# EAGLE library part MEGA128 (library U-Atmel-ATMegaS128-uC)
MICROCONTROLLER 128 Kbytes FLASH 4 Kbytes SRAM 4 Kbytes EEPROM DUAL USART 8-channel 10 bit ADC Source: avr.lbr
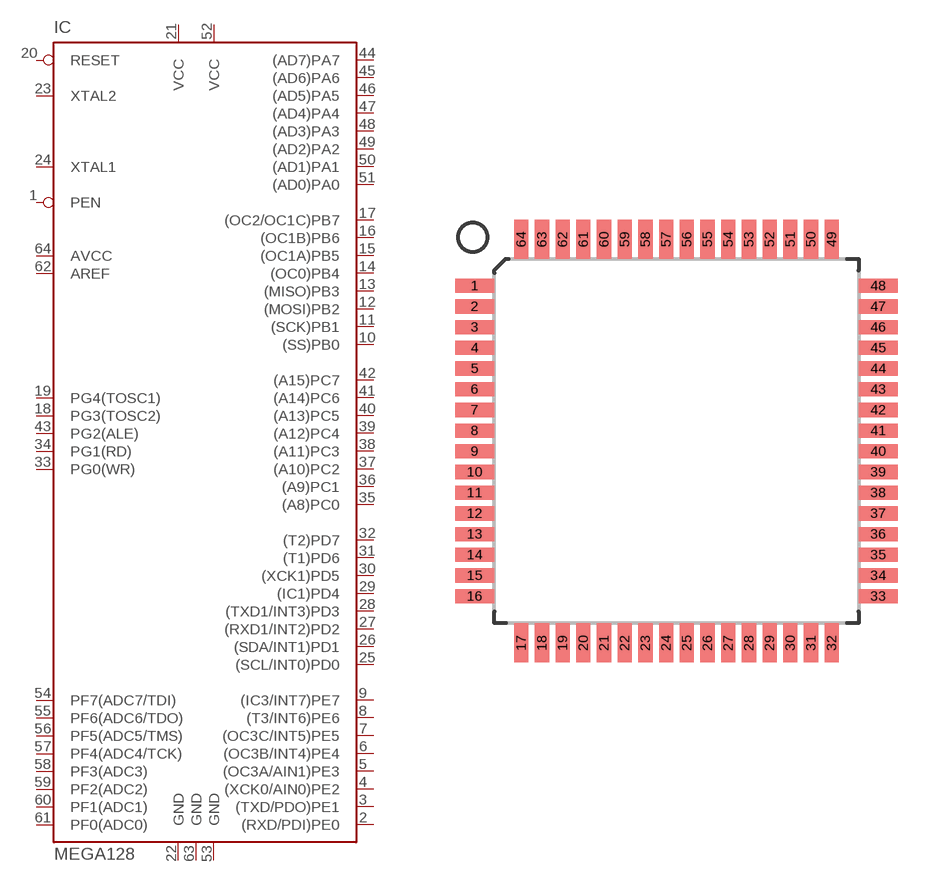
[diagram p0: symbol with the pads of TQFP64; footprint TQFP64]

Designator prefix IC

## MEGA128-A (MPN: ATMEGA128-16AU; OC_FARNELL: 9171118; OC_NEWARK: 95K7364)  [TQFP64]
1  PEN  in
2  (RXD/PDI)PE0
3  (TXD/PDO)PE1
4  (XCK0/AIN0)PE2
5  (OC3A/AIN1)PE3
6  (OC3B/INT4)PE4
7  (OC3C/INT5)PE5
8  (T3/INT6)PE6
9  (IC3/INT7)PE7
10  (SS)PB0
11  (SCK)PB1
12  (MOSI)PB2
13  (MISO)PB3
14  (OC0)PB4
15  (OC1A)PB5
16  (OC1B)PB6
17  (OC2/OC1C)PB7
18  PG3(TOSC2)
19  PG4(TOSC1)
20  RESET  in
21  VCC  pwr
22  GND  pwr
23  XTAL2  pas
24  XTAL1  pas
25  (SCL/INT0)PD0
26  (SDA/INT1)PD1
27  (RXD1/INT2)PD2
28  (TXD1/INT3)PD3
29  (IC1)PD4
30  (XCK1)PD5
31  (T1)PD6
32  (T2)PD7
33  PG0(WR)
34  PG1(RD)
35  (A8)PC0
36  (A9)PC1
37  (A10)PC2
38  (A11)PC3
39  (A12)PC4
40  (A13)PC5
41  (A14)PC6
42  (A15)PC7
43  PG2(ALE)
44  (AD7)PA7
45  (AD6)PA6
46  (AD5)PA5
47  (AD4)PA4
48  (AD3)PA3
49  (AD2)PA2
50  (AD1)PA1
51  (AD0)PA0
52  VCC  pwr
53  GND  pwr
54  PF7(ADC7/TDI)
55  PF6(ADC6/TDO)
56  PF5(ADC5/TMS)
57  PF4(ADC4/TCK)
58  PF3(ADC3)
59  PF2(ADC2)
60  PF1(ADC1)
61  PF0(ADC0)
62  AREF  pas
63  GND  pwr
64  AVCC  pwr

## Footprint TQFP64 (pad centres in mm)
Thin Plasic Quad Flat Package Updated from atml.lbr 17.01.2005 alf@cadsoft.de
smd 1.5 x 0.55: 1 -7.8,6; 2 -7.8,5.2; 3 -7.8,4.4; 4 -7.8,3.6; 5 -7.8,2.8; 6 -7.8,2; 7 -7.8,1.2; 8 -7.8,0.4; 9 -7.8,-0.4; 10 -7.8,-1.2; 11 -7.8,-2; 12 -7.8,-2.8; 13 -7.8,-3.6; 14 -7.8,-4.4; 15 -7.8,-5.2; 16 -7.8,-6; 33 7.8,-6; 34 7.8,-5.2; 35 7.8,-4.4; 36 7.8,-3.6; 37 7.8,-2.8; 38 7.8,-2; 39 7.8,-1.2; 40 7.8,-0.4; 41 7.8,0.4; 42 7.8,1.2; 43 7.8,2; 44 7.8,2.8; 45 7.8,3.6; 46 7.8,4.4; 47 7.8,5.2; 48 7.8,6
smd 0.55 x 1.5: 17 -6,-7.8; 18 -5.2,-7.8; 19 -4.4,-7.8; 20 -3.6,-7.8; 21 -2.8,-7.8; 22 -2,-7.8; 23 -1.2,-7.8; 24 -0.4,-7.8; 25 0.4,-7.8; 26 1.2,-7.8; 27 2,-7.8; 28 2.8,-7.8; 29 3.6,-7.8; 30 4.4,-7.8; 31 5.2,-7.8; 32 6,-7.8; 49 6,7.8; 50 5.2,7.8; 51 4.4,7.8; 52 3.6,7.8; 53 2.8,7.8; 54 2,7.8; 55 1.2,7.8; 56 0.4,7.8; 57 -0.4,7.8; 58 -1.2,7.8; 59 -2,7.8; 60 -2.8,7.8; 61 -3.6,7.8; 62 -4.4,7.8; 63 -5.2,7.8; 64 -6,7.8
